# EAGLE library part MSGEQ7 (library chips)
A CMOS spectrum analyzer
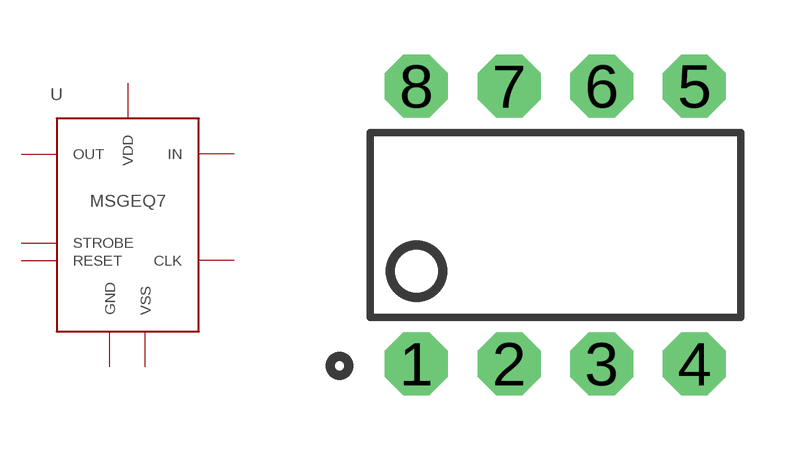
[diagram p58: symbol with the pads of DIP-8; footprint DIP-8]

Designator prefix U

## MSGEQ7 (DIGIKEY: 1568-1335-ND; MANUFACTURER: Sparkfun Electronics; MPN: COM-10468)  [DIP-8]
1  VDD
2  VSS
3  OUT
4  STROBE
5  IN
6  GND
7  RESET
8  CLK

## Footprint DIP-8 (pad centres in mm)
drill 0.813 pad 1.727 octagon: 1 -3.81,-3.81; 2 -1.27,-3.81; 3 1.27,-3.81; 4 3.81,-3.81; 5 3.81,3.81; 6 1.27,3.81; 7 -1.27,3.81; 8 -3.81,3.81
